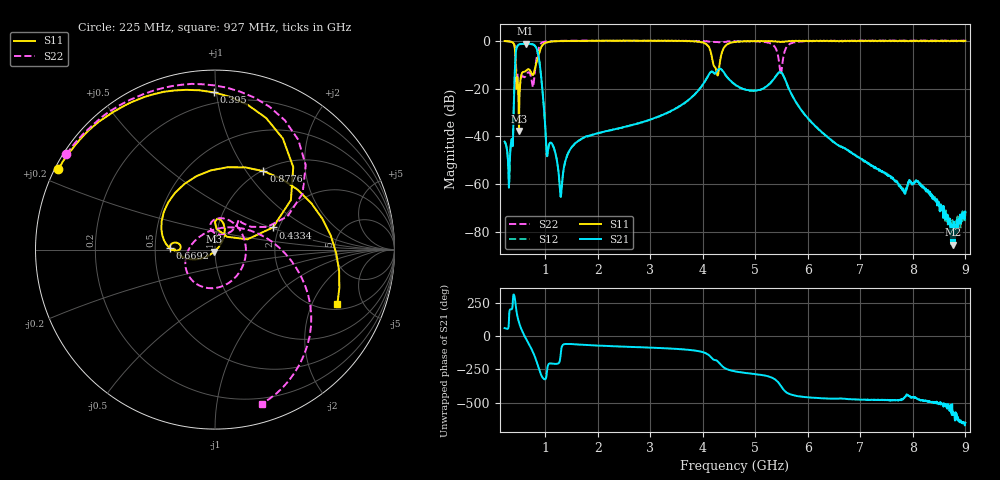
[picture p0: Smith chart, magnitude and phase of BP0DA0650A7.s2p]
!Agilent Technologies,E8358A,US40260310,A.06.04.32
!Agilent E8358A: A.06.04.32
!Date: Friday, June 14, 2019 23:30:36
!Correction: S11(Full 2 Port(1,2)) S21(Full 2 Port(1,2)) S12(Full 2 Port(1,2)) S22(Full 2 Port(1,2))
!S2P File: Measurements: S11, S21, S12, S22:
# Hz S  dB  R 50
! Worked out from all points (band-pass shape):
!   1601 points, 225 MHz to 9 GHz, reference 50 ohm
!   highest |S21| = -1.28 dB at 625.4 MHz (marker M1); lowest = -85.3 dB at 8.77 GHz (marker M2)
!   |S21| within 3 dB of the highest: 441.5 MHz to 849 MHz (407.5 MHz wide, 63.2 % of centre)
!   lowest |S11| = -37.7 dB at 499.2 MHz (marker M3), VSWR 1.03, Z = 49.5 - j1.21 ohm
!   |S11| at or under -10 dB: 434.2 MHz to 821 MHz (386.8 MHz wide, 61.6 % of centre); 4.202 GHz to 4.318 GHz (116.1 MHz wide, 2.73 % of centre)
!   |S22| runs from -21.3 to 0.1 dB; largest |S21 - S12| = 0.0076
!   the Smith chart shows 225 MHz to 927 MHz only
!   S11 on the Smith chart (normalised r, x): 225 MHz: 0.01, +0.24; 395 MHz: 0.13, +0.98; 433.4 MHz: 1.86, +0.52; 669.2 MHz: 0.60, +0.01; 877.6 MHz: 1.02, +1.21; 927 MHz: 2.28, -3.14
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2.25e8  -0.17 152.9  -42.19 58.8  -42.23 58.7  -0.15 147.3
3.346875e8  -0.41 126.6  -45.68 -160.2  -45.73 -160.3  -0.39 117.2
3.950156e8  -1.15 90.4  -31.33 -49.4  -31.40 -49.3  -1.00 81.0
4.334062e8  -9.23 20.9  -6.27 -119.6  -6.33 -119.5  -7.06 24.6
4.992188e8  -37.73 -110.1  -1.59 100.8  -1.65 100.9  -21.28 76.0
6.253594e8  -12.69 -179.6  -1.28 -15.7  -1.34 -15.7  -14.82 -34.3
6.692344e8  -11.99 178.0  -1.35 -47.8  -1.40 -47.8  -13.32 -94.1
8.776406e8  -5.78 58.3  -7.22 114.6  -7.29 114.5  -2.93 -42.3
9.27e8  -2.54 -24.0  -16.34 62.5  -16.39 62.6  -0.95 -73.1
1.031203e9  -0.72 -92.7  -48.18 91.6  -48.31 91.7  -0.32 -105.9
1.288969e9  -0.20 -135.6  -64.95 -152.8  -64.82 -152.1  -0.11 -135.7
1.689328e9  -0.11 -155.6  -41.00 -65.3  -41.06 -65.2  0.01 -151.3
3.153656e9  -0.03 -179.3  -31.68 -90.4  -31.72 -90.2  -0.02 -177.3
4.096969e9  -2.15 128.9  -14.89 -138.3  -14.96 -138.4  -0.41 163.2
4.305375e9  -12.08 -29.1  -11.82 160.5  -11.94 161.1  -0.69 161.0
4.6125e9  -0.60 -153.6  -18.31 94.0  -18.38 94.4  -0.23 154.4
5.451609e9  -0.44 178.4  -13.22 3.9  -13.35 4.3  -9.01 43.7
5.649047e9  -0.15 176.9  -20.52 -75.6  -20.59 -74.9  -1.43 -175.1
6.076828e9  -0.17 171.2  -34.28 -102.8  -34.35 -103.0  -0.22 150.9
7.541156e9  -0.05 155.7  -56.33 -121.4  -56.32 -121.1  -0.08 132.7
8.769656e9  -0.23 144.3  -85.25 125.6  -80.30 164.9  -0.04 125.7
9e9  -0.05 142.0  -71.59 68.6  -71.23 61.5  -0.08 125.2
